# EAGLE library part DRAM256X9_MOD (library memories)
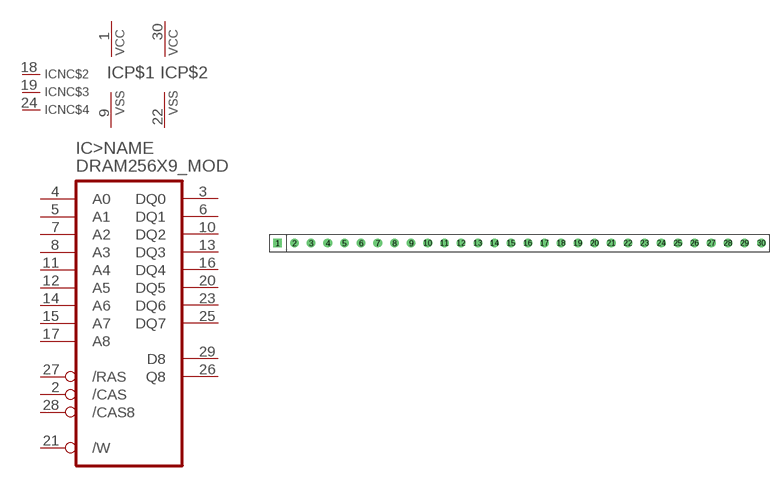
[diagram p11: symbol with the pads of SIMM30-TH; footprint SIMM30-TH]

Designator prefix IC; gates >NAME=DRAM256KX9 NC$2=NC NC$3=NC NC$4=NC P$1=VCCVSS P$2=VCCVSS

## DRAM256X9_MOD  [SIMM30-TH]
1  P$1:VCC  pwr
2  >NAME:/CAS  in
3  >NAME:DQ0
4  >NAME:A0  in
5  >NAME:A1  in
6  >NAME:DQ1
7  >NAME:A2  in
8  >NAME:A3  in
9  P$1:VSS  pwr
10  >NAME:DQ2
11  >NAME:A4  in
12  >NAME:A5  in
13  >NAME:DQ3
14  >NAME:A6  in
15  >NAME:A7  in
16  >NAME:DQ4
17  >NAME:A8  in
18  NC$2:NC  nc
19  NC$3:NC  nc
20  >NAME:DQ5
21  >NAME:/W  in
22  P$2:VSS  pwr
23  >NAME:DQ6
24  NC$4:NC  nc
25  >NAME:DQ7
26  >NAME:Q8  out
27  >NAME:/RAS  in
28  >NAME:/CAS8  in
29  >NAME:D8  in
30  P$2:VCC  pwr

## Footprint SIMM30-TH (pad centres in mm)
drill 0.8 square: 1 0,0
drill 0.8: 2 2.54,0; 3 5.08,0; 4 7.62,0; 5 10.16,0; 6 12.7,0; 7 15.24,0; 8 17.78,0; 9 20.32,0; 10 22.86,0; 11 25.4,0; 12 27.94,0; 13 30.48,0; 14 33.02,0; 15 35.56,0; 16 38.1,0; 17 40.64,0; 18 43.18,0; 19 45.72,0; 20 48.26,0; 21 50.8,0; 22 53.34,0; 23 55.88,0; 24 58.42,0; 25 60.96,0; 26 63.5,0; 27 66.04,0; 28 68.58,0; 29 71.12,0; 30 73.66,0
